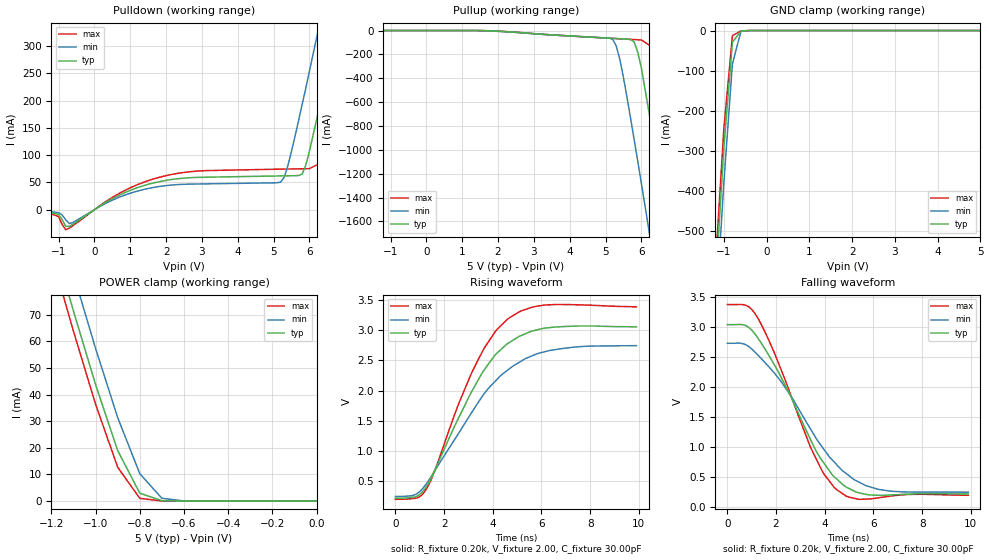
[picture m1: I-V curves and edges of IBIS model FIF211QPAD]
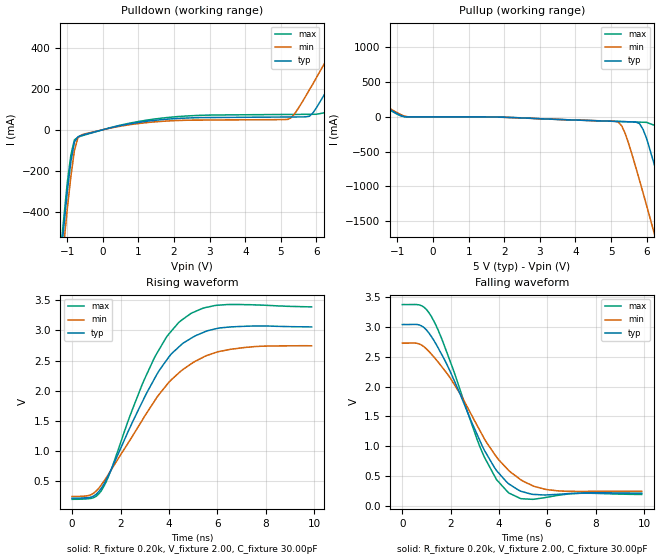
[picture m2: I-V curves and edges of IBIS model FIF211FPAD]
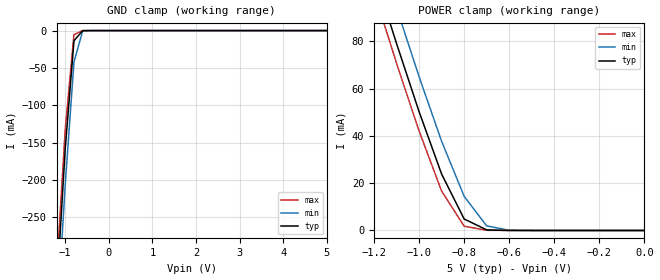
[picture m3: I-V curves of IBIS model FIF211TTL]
| IBIS file idt72801.ibs created by s2ibis2 version 1.1
| North Carolina State University Electronics Research Laboratory  1995
[IBIS ver]   2.1
[File name]   idt72801.ibs
[File Rev]   1.0
[Date]   12/19/97
[Source]   Integrated Device Technology, Inc.
[Notes]   1. Temperatures: typ=25C, min=70C, max=0C 2. Cemos8_5v
   process. 3. Ramp rates based on 50 ohm load.
[Copyright]   Copyright 1997, Integrated Device Technology, Inc.
|   Component idt72801
[Component]   idt72801
[Manufacturer]   Integrated Device Technology
[Package]
| variable   typ   min   max
R_pkg   0.75   0.60   0.90
L_pkg   8.10nH   8.30nH   9.90nH
C_pkg   0.53pF   0.46pF   0.60pF
[Pin]  signal_name   model_name   R_pin   L_pin   C_pin
1   QA1   FIF211QPAD
2   QA2   FIF211QPAD
3   QA3   FIF211QPAD
4   QA4   FIF211QPAD
5   QA5   FIF211QPAD
6   QA6   FIF211QPAD
7   QA7   FIF211QPAD
8   QA8   FIF211QPAD
9   VCC   POWER
10   WENA2   FIF211TTL
11   WCLKA   FIF211TTL
12   WENAL1   FIF211TTL
13   RSAL   FIF211TTL
14   DA8   FIF211TTL
15   DA7   FIF211TTL
16   DA6   FIF211TTL
17   DA5   FIF211TTL
18   DA4   FIF211TTL
19   DA3   FIF211TTL
20   DA2   FIF211TTL
21   DA1   FIF211TTL
22   DA0   FIF211TTL
23   PAFAL   FIF211FPAD
24   PAEAL   FIF211FPAD
25   WENB2   FIF211TTL
26   WCLKB   FIF211TTL
27   WENBL1   FIF211TTL
28   RSBL   FIF211TTL
29   DB8   FIF211TTL
30   DB7   FIF211TTL
31   DB6   FIF211TTL
32   DB5   FIF211TTL
33   DB4   FIF211TTL
34   DB3   FIF211TTL
35   DB2   FIF211TTL
36   DB1   FIF211TTL
37   DB0   FIF211TTL
38   PAFBL   FIF211FPAD
39   PAEBL   FIF211FPAD
40   VCC   POWER
41   GND   GND
42   RENBL1   FIF211TTL
43   RCLKB   FIF211TTL
44   RENBL2   FIF211TTL
45   OEBL   FIF211TTL
46   EFBL   FIF211FPAD
47   FFBL   FIF211FPAD
48   QB0   FIF211QPAD
49   QB1   FIF211QPAD
50   QB2   FIF211QPAD
51   QB3   FIF211QPAD
52   QB4   FIF211QPAD
53   QB5   FIF211QPAD
54   QB6   FIF211QPAD
55   QB7   FIF211QPAD
56   QB8   FIF211QPAD
57   GND   GND
58   RENAL1   FIF211TTL
59   RCLKA   FIF211TTL
60   RENAL2   FIF211TTL
61   OEAL   FIF211TTL
62   EFAL   FIF211FPAD
63   FFAL   FIF211FPAD
64   QA0   FIF211QPAD
| Models and submodels in the file (3): FIF211QPAD (3-state), FIF211FPAD (Output), FIF211TTL (Input)
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| FIN  FIN   dummy_model
| QIN  QIN   dummy_model
| QOEL QOEL   dummy_model
|   Model FIF211QPAD
[Model]   FIF211QPAD
Model_type   3-state
Polarity   Non-Inverting
Enable   Active-Low
Vmeas =  1.500V
C_comp   3.00pF   NA   NA
[Temperature Range]   25.00   70.00   0.000
[Voltage Range]   5.00V   4.50V   5.50V
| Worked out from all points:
|   slope of the pulldown table from 0 to 0.75 V, typ, clamps not added: 26.4 ohm
|   GND clamp passes 1 mA (typ) near -0.58 V on its own axis
|   POWER clamp passes 1 mA (typ) near -0.73 V on its own axis
|   rising waveform, R_fixture 0.20k, V_fixture 2.00, C_fixture 30.00pF: 20-80 % time 2.17ns typ, 2.58ns min, 1.96ns max; typ from 0.212 V to 3.06 V
|   falling waveform, R_fixture 0.20k, V_fixture 2.00, C_fixture 30.00pF: 20-80 % time 2.1ns typ, 2.47ns min, 1.87ns max; typ from 3.04 V to 0.213 V
[Pulldown]
| voltage   I(typ)   I(min)   I(max)
-5V       0A         0A         0A
-1.4V     -3mA       -2mA       -2.6mA
-800mV    -30.42mA   -18.6mA    -36.69mA
1.7V      49.86mA    41.4mA     57.4mA
5.2V      62.01mA    50.61mA    74.43mA
5.4V      62.22mA    81.07mA    74.66mA
5.8V      65.63mA    194mA      75.11mA
6V        107mA      254mA      75.33mA
6.4V      223mA      376mA      88.46mA
6.8V      345mA      500mA      198mA
7.2V      469mA      624mA      320mA
10V       1.346A     1.502A     1.195A
[Pullup]
| voltage   I(typ)   I(min)   I(max)
-5V       0A         0A         0A
1.5V      -479uA     -1.046mA   -164uA
5.2V      -65.7mA    -73.36mA   -65.97mA
5.3V      -67.33mA   -129mA     -67.59mA
5.4V      -68.96mA   -242mA     -69.22mA
5.8V      -96.18mA   -914mA     -75.69mA
6V        -312mA     -1.279A    -78.93mA
6.4V      -1.008A    -2.023A    -157mA
6.8V      -1.75A     -2.776A    -778mA
7.2V      -2.503A    -3.534A    -1.516A
7.6V      -3.262A    -4.295A    -2.268A
10V       -7.849A    -8.885A    -6.849A
[GND_clamp]
| voltage   I(typ)   I(min)   I(max)
-5V       -7.849A    -7.926A    -7.807A
-1.2V     -640mA     -729mA     -591mA
-1V       -293mA     -381mA     -246mA
-800mV    -29.29mA   -83.51mA   -12.91mA
-600mV    -1.086mA   -1.828mA   -995uA
-400mV    -11.7nA    -1.657uA   -4.457nA
5V        50nA       1.239uA    50nA
[POWER_clamp]
| voltage   I(typ)   I(min)   I(max)
-5V       1.28A      1.292A     1.273A
-1.2V     100mA      114mA      92.56mA
-1.1V     71.31mA    85.16mA    63.76mA
-1V       43.75mA    57.31mA    36.34mA
-900mV    18.98mA    31.36mA    12.72mA
-800mV    2.991mA    10.3mA     1.049mA
-700mV    169uA      1.084mA    64.47uA
-600mV    6.517uA    77.91uA    260nA
0V        50nA       45nA       55nA
[Ramp]
| variable   typ   min   max
dV/dt_r   1.00/1.26n   0.85/1.56n   1.15/1.09n
dV/dt_f   1.67/2.34n   1.36/2.84n   1.96/2.00n
R_load = 50.00
[Rising Waveform]
R_fixture = 0.20k
V_fixture = 2.00
C_fixture = 30.00pF
R_dut = 0.75
L_dut = 8.10nH
C_dut = 0.53pF
| time   V(typ)   V(min)   V(max)
0s        212mV      240mV      193mV
800ps     232mV      269mV      209mV
1.3ns     418mV      465mV      383mV
2.6ns     1.55V      1.292V     1.78V
3.2ns     2.031V     1.677V     2.351V
4.1ns     2.594V     2.155V     2.979V
4.6ns     2.779V     2.337V     3.185V
5.2ns     2.92V      2.497V     3.328V
6.3ns     3.045V     2.663V     3.425V
9.9ns     3.059V     2.746V     3.391V
[Falling Waveform]
R_fixture = 0.20k
V_fixture = 2.00
C_fixture = 30.00pF
R_dut = 0.75
L_dut = 8.10nH
C_dut = 0.53pF
| time   V(typ)   V(min)   V(max)
0s        3.045V     2.733V     3.38V
800ps     3.02V      2.7V       3.36V
1.2ns     2.853V     2.56V      3.189V
2.2ns     2.172V     2.099V     2.301V
3.5ns     1.051V     1.244V     923mV
3.9ns     767mV      997mV      592mV
4.5ns     461mV      699mV      283mV
5.3ns     244mV      434mV      133mV
6.2ns     192mV      291mV      149mV
9.9ns     213mV      243mV      192mV
|   Model FIF211FPAD
[Model]   FIF211FPAD
Model_type   Output
Vmeas =  1.500V
C_comp   3.00pF   NA   NA
[Temperature Range]   25.00   70.00   0.000
[Voltage Range]   5.00V   4.50V   5.50V
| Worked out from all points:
|   slope of the pulldown table from 0 to 0.75 V, typ, clamps not added: 26.4 ohm
|   rising waveform, R_fixture 0.20k, V_fixture 2.00, C_fixture 30.00pF: 20-80 % time 2.16ns typ, 2.57ns min, 1.95ns max; typ from 0.212 V to 3.06 V
|   falling waveform, R_fixture 0.20k, V_fixture 2.00, C_fixture 30.00pF: 20-80 % time 1.9ns typ, 2.24ns min, 1.69ns max; typ from 3.04 V to 0.212 V
[Pulldown]
| voltage   I(typ)   I(min)   I(max)
-5V       -7.849A    -7.926A    -7.807A
-1.4V     -1.006A    -1.093A    -958mA
-1V       -302mA     -386mA     -259mA
-800mV    -59.72mA   -102mA     -49.6mA
-600mV    -27.75mA   -25.16mA   -30.34mA
5.2V      62.01mA    50.61mA    74.43mA
5.8V      65.63mA    194mA      75.11mA
6.4V      223mA      376mA      88.46mA
6.8V      345mA      500mA      198mA
7.2V      469mA      624mA      320mA
8V        718mA      874mA      568mA
10V       1.346A     1.502A     1.195A
[Pullup]
| voltage   I(typ)   I(min)   I(max)
-5V       1.28A      1.292A     1.273A
-1.4V     160mA      173mA      152mA
-800mV    2.991mA    10.3mA     1.049mA
5.2V      -65.7mA    -73.36mA   -65.97mA
5.4V      -68.96mA   -242mA     -69.22mA
5.8V      -96.18mA   -914mA     -75.69mA
6V        -312mA     -1.279A    -78.93mA
6.4V      -1.008A    -2.023A    -157mA
6.8V      -1.75A     -2.776A    -778mA
7.2V      -2.503A    -3.534A    -1.516A
7.6V      -3.262A    -4.295A    -2.268A
10V       -7.849A    -8.885A    -6.849A
[Ramp]
| variable   typ   min   max
dV/dt_r   1.00/1.25n   0.85/1.55n   1.15/1.07n
dV/dt_f   1.67/1.85n   1.36/2.28n   1.96/1.61n
R_load = 50.00
[Rising Waveform]
R_fixture = 0.20k
V_fixture = 2.00
C_fixture = 30.00pF
R_dut = 0.75
L_dut = 8.10nH
C_dut = 0.53pF
| time   V(typ)   V(min)   V(max)
0s        212mV      240mV      193mV
800ps     231mV      273mV      210mV
1.2ns     371mV      429mV      331mV
1.6ns     674mV      673mV      670mV
2.9ns     1.812V     1.509V     2.106V
3.4ns     2.194V     1.823V     2.545V
3.9ns     2.503V     2.089V     2.889V
4.5ns     2.758V     2.326V     3.163V
6.1ns     3.041V     2.652V     3.421V
9.9ns     3.058V     2.745V     3.391V
[Falling Waveform]
R_fixture = 0.20k
V_fixture = 2.00
C_fixture = 30.00pF
R_dut = 0.75
L_dut = 8.10nH
C_dut = 0.53pF
| time   V(typ)   V(min)   V(max)
0s        3.045V     2.733V     3.38V
800ps     3.021V     2.699V     3.36V
1.2ns     2.844V     2.548V     3.181V
2ns       2.237V     2.134V     2.403V
3.3ns     1.009V     1.194V     902mV
3.9ns     588mV      816mV      436mV
4.4ns     368mV      593mV      215mV
4.9ns     244mV      436mV      119mV
6ns       183mV      270mV      144mV
9.9ns     212mV      242mV      190mV
|   Model FIF211TTL
[Model]   FIF211TTL
Model_type   Input
Vinl =  0.000V
Vinh =  3.000V
Vmeas =  1.500V
C_comp   3.00pF   NA   NA
[Temperature Range]   25.00   70.00   0.000
[Voltage Range]   5.00V   4.50V   5.50V
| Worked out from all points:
|   GND clamp passes 1 mA (typ) near -0.61 V on its own axis
|   POWER clamp passes 1 mA (typ) near -0.72 V on its own axis
[GND_clamp]
| voltage   I(typ)   I(min)   I(max)
-5V       -4.391A    -4.433A    -4.368A
-1.2V     -352mA     -401mA     -325mA
-1V       -158mA     -206mA     -132mA
-800mV    -13.65mA   -42.02mA   -5.426mA
-600mV    -95.68uA   -488uA     -19.8uA
5V        50nA       2.529uA    50nA
[POWER_clamp]
| voltage   I(typ)   I(min)   I(max)
-5V       1.33A      1.343A     1.323A
-1.2V     109mA      124mA      101mA
-1.1V     79.07mA    94.22mA    70.74mA
-1V       50.25mA    65.05mA    42.12mA
-900mV    23.87mA    37.74mA    16.67mA
-800mV    4.863mA    14.45mA    1.814mA
-700mV    253uA      1.929mA    79.02uA
-600mV    7.842uA    115uA      476nA
0V        50nA       45nA       55nA
